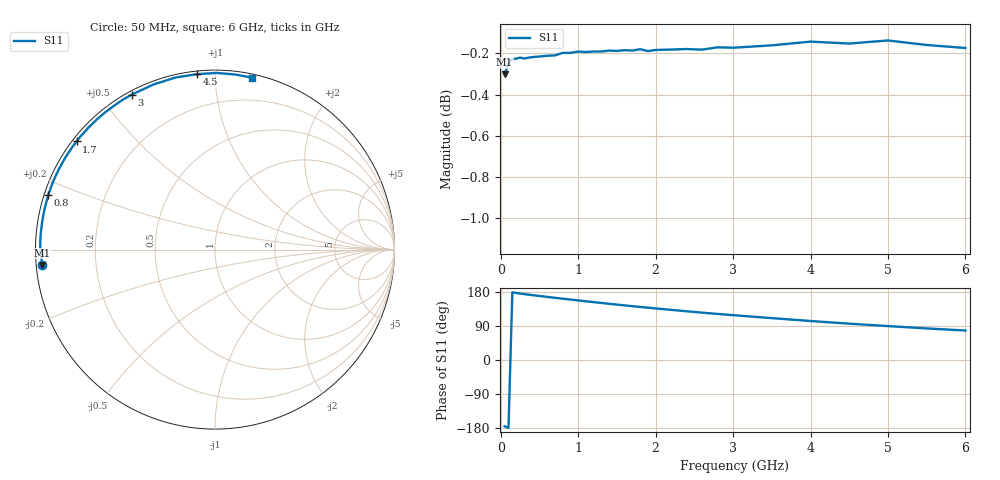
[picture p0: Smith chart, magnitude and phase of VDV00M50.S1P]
! Infineon Technologies  Discrete & RF Semiconductors
! BBY 55-03
! Si Tuning Diode in SOD323
! VR =
! S-Parameters:  June  1999
# GHz  S  MA  R  50
!  f  S11
! GHz  MAG  ANG
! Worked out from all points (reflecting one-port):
!   34 points, 50 MHz to 6 GHz, reference 50 ohm
!   lowest |S11| = -0.3 dB at 50 MHz (marker M1), VSWR 57.50, Z = 0.871 - j2.23 ohm
!   phase of S11 starts at -175 deg and turns -107 deg over the sweep
!   S11 on the Smith chart (normalised r, x): 50 MHz: 0.02, -0.04; 800 MHz: 0.01, +0.16; 1.7 GHz: 0.01, +0.34; 3 GHz: 0.01, +0.60; 4.5 GHz: 0.02, +0.90; 6 GHz: 0.03, +1.24
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0.05  0.9658 -174.9
0.1  0.9722 -179.2
0.15  0.9742 178.6
0.2  0.9744 176.9
0.3  0.9745 174.0
0.4  0.9752 171.4
0.5  0.9756 169.0
0.6  0.976 166.5
0.8  0.9776 161.8
1  0.9783 157.2
1.1  0.978 154.9
1.2  0.9783 152.7
1.4  0.9788 148.3
1.6  0.979 144.1
1.7  0.9788 142.0
1.8  0.9796 140.0
2  0.9791 136.1
2.2  0.9794 132.3
2.4  0.9797 128.6
2.6  0.9793 125.0
2.8  0.9806 121.6
3  0.9804 118.3
3.5  0.9817 110.5
4  0.9837 102.9
4.5  0.9827 95.9
5  0.9844 89.5
5.5  0.9819 83.3
6  0.9802 77.8
